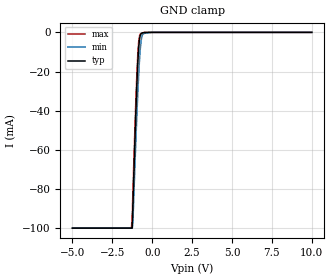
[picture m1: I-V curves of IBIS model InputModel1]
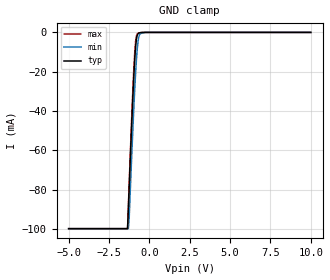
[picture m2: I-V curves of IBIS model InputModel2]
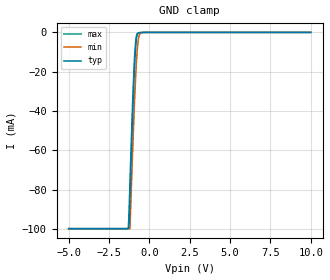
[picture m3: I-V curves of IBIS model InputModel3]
[IBIS Ver]   2.1
[File name]   ef008sa5.ibs   | e= TSOP f= Reverse Pinout,
|   | f0008sa= abbr chip name, 5= 5V Vcc
[File Rev]   2.00
[Date]   23-February-96
[Source]   File generated from lab measurements at Intel Corporation
[Notes]   Rev 2.00 All data was replaced by actual measurements
   performed in a lab.
[Disclaimer] INTEL DEVELOPER'S SOFTWARE LICENSE AGREEMENT
| BY USING THIS SOFTWARE, YOU ARE AGREEING TO BE BOUND
| BY THE TERMS OF THIS AGREEMENT.  DO NOT USE THE SOFTWARE
| UNTIL YOU HAVE CAREFULLY READ AND AGREED TO THE FOLLOWING
| TERMS AND CONDITIONS.  IF YOU DO NOT AGREE TO THE TERMS
| OF THIS AGREEMENT, PROMPTLY RETURN THE SOFTWARE PACKAGE
| AND ANY ACCOMPANYING ITEMS.
| IF YOU USE THIS SOFTWARE, YOU WILL BE BOUND BY THE TERMS
| OF THIS AGREEMENT
| LICENSE: Intel Corporation ("Intel") grants you the non-exclusive right
| to use the enclosed software program ("Software").  You will not use,
| copy, modify, rent, sell or transfer the Software or any portion
| thereof, except as provided in this Agreement.
| System OEM Developers may:
| 1.   Copy the Software for support, backup or archival purposes;
| 2.   Install, use, or distribute Intel owned Software in object code
|   only;
| 3.   Modify and/or use Software source code that Intel directly makes
|   available to you as an OEM Developer;
| 4.   Install, use, modify, distribute, and/or make or have made
|   derivatives ("Derivatives") of Intel owned Software under the
|   terms and conditions in this Agreement, ONLY if you are a System
|   OEM Developer and NOT an end-user.
| RESTRICTIONS:
| YOU WILL NOT:
| 1.   Copy the Software, in whole or in part, except as provided for
|   in this Agreement;
| 2.   Decompile or reverse engineer any Software provided in object
|   code format;
| 3.   Distribute any Software or Derivative code to any end-users,
|   unless approved by Intel in a prior writing.
| TRANSFER: You may transfer the Software to another OEM
| Developer if the receiving party agrees to the terms of this
| Agreement at the sole risk of any receiving party.
| OWNERSHIP AND COPYRIGHT OF SOFTWARE:
| Title to the Software and all copies thereof remain with Intel
| or its vendors.  The Software is copyrighted and is protected by
| United States and international copyright laws.  You will not
| remove the copyright notice from the Software.  You agree to
| prevent any unauthorized copying of the Software.
| DERIVATIVE WORK: OEM Developers that make or have made
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[Copyright]   Copyright 1996, Intel Corporation, All Rights Reserved
[Component]   F28F008SA   | 40-lead TSOP package, 28F008SA
[Manufacturer]  Intel   | Boot Block (tm)
|   | operating in 5V Vcc range
[Package]
|The following values apply for the leadframe.
|Variable   typ   min   max
R_pkg   135m   126m   144m
L_pkg   3.95nH   3.62nH   4.28nH
C_pkg   0.39pF   0.38pF   0.40pF
|*****************************Pin Definitions**********************************
[Pin]   signal_name   model_name   R_pin   L_pin   C_pin
  1   NC   InputModel5
  2   NC   InputModel5
  3   WE#   InputModel3
  4   OE#   InputModel3
  5   RYBY#   RYBYOutput
  6   DQ7   InputOutput
  7   DQ6   InputOutput
  8   DQ5   InputOutput
  9   DQ4   InputOutput
 10   VCC   POWER
 11   GND   GND
 12   GND   GND
 13   DQ3   InputOutput
 14   DQ2   InputOutput
 15   DQ1   InputOutput
 16   DQ0   InputOutput
 17   A00   InputModel1
 18   A01   InputModel1
 19   A02   InputModel1
 20   A03   InputModel1
 21   A04   InputModel2
 22   A05   InputModel2
 23   A06   InputModel2
 24   A07   InputModel2
 25   A08   InputModel2
 26   A09   InputModel2
 27   A10   InputModel2
 28   A11   InputModel2
 29   RP#   InputModel4
 30   VPP   POWER
 31   VCC   POWER
 32   CE#   InputModel3
 33   A12   InputModel2
 34   A13   InputModel2
 35   A14   InputModel2
 36   A15   InputModel2
 37   A16   InputModel2
 38   A17   InputModel2
 39   A18   InputModel2
 40   A19   InputModel2
|**********************Input Model 5***************************************
[Model]   InputModel5
Model_type   Input
|   For NC pins
Vinl = 0.8V
Vinh = 2.0V
| Variable   typ   min   max
C_comp   5.61p   NA   7.6p
[Voltage Range]   5.0V   4.5V   5.5V
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| Models and submodels in the file (7): InputModel1 (Input), InputModel2 (Input), InputModel3 (Input), InputModel4 (Input), InputModel5 (Input), InputOutput (I/O), RYBYOutput (Output)
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|**************************Input Model 1***************************************
[Model]   InputModel1
Model_type   Input
|   For A[3:0]
Vinl = 0.8V
Vinh = 2.0V
| Variable   typ   min   max
C_comp   5.61p   NA   7.6p
[Voltage Range]   5.0V   4.5V   5.5V
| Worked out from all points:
|   GND clamp passes 1 mA (typ) near -0.72 V on its own axis
[GND_clamp]
|Voltage I(typ)   I(min)   I(max)
-5V       -99.85mA   -99.84mA   -99.85mA
-1.3V     -99.85mA   -99.84mA   -99.85mA
-1.25V    -99.83mA   -99.84mA   -92.56mA
-1.2V     -85.91mA   -94.75mA   -78.96mA
-1.05V    -46.93mA   -60.78mA   -40.45mA
-950mV    -24.37mA   -39.94mA   -18.85mA
-850mV    -8.175mA   -22.06mA   -4.862mA
-800mV    -3.667mA   -14.55mA   -1.917mA
-700mV    -717.5uA   -4.645mA   -522.5uA
-600mV    -274uA     -1.047mA   -226.9uA
0V        0A         0A         0A
10V       0A         0A         0A
[POWER_clamp]
| Input buffer circuits of this product do not intrinsically
| require a [POWER_clamp] definition.  This zero current
| [POWER_clamp] is provided for compatibility with some ibis
| parsers.
|   Voltage  I(typ)   I(min)   I(max)
-5V       0A         0A         0A
-4.75V    0A         0A         0A
9.75V     0A         0A         0A
10V       0A         0A         0A
|**********************Input Model 2************************************
[Model]   InputModel2
Model_type   Input
|   For A[19:4]
Vinl = 0.8V
Vinh = 2.0V
| Variable   typ   min   max
C_comp   5.61p   NA   7.6p
[Voltage Range]   5.0V   4.5V   5.5V
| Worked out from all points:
|   GND clamp passes 1 mA (typ) near -0.73 V on its own axis
[GND_clamp]
|Voltage I(typ)   I(min)   I(max)
-5V       -99.84mA   -99.84mA   -99.84mA
-1.35V    -99.84mA   -99.84mA   -99.84mA
-1.3V     -90.06mA   -99.84mA   -88.39mA
-1.25V    -79.28mA   -94.68mA   -77.04mA
-1.1V     -48.07mA   -64.47mA   -44.59mA
-950mV    -20.49mA   -36.5mA    -16.5mA
-850mV    -7.244mA   -20.62mA   -4.445mA
-750mV    -1.356mA   -8.439mA   -748.5uA
-700mV    -613.5uA   -4.588mA   -433.7uA
-600mV    -217.8uA   -1.014mA   -177.9uA
-250mV    0A         0A         0A
10V       0A         0A         0A
[POWER_clamp]
| Input buffer circuits of this product do not intrinsically
| require a [POWER_clamp] definition.  This zero current
| [POWER_clamp] is provided for compatibility with some ibis
| parsers.
|   Voltage  I(typ)   I(min)   I(max)
-5V       0A         0A         0A
-4.75V    0A         0A         0A
9.75V     0A         0A         0A
10V       0A         0A         0A
|*********************Input Model 3**************************************
[Model]   InputModel3
Model_type   Input
|   For WE#, OE# & CE#
Vinl = 0.8V
Vinh = 2.0V
| Variable   typ   min   max
C_comp   5.61p   NA   7.6p
[Voltage Range]   5.0V   4.5V   5.5V
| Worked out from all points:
|   GND clamp passes 1 mA (typ) near -0.73 V on its own axis
[GND_clamp]
|Voltage I(typ)   I(min)   I(max)
-5V       -99.85mA   -99.84mA   -99.85mA
-1.3V     -99.85mA   -99.84mA   -99.85mA
-1.25V    -96.72mA   -99.84mA   -89.03mA
-1.2V     -83.27mA   -99.84mA   -75.92mA
-1.05V    -45.34mA   -63.96mA   -38.88mA
-950mV    -23.44mA   -41.82mA   -18.03mA
-900mV    -14.49mA   -31.8mA    -10.01mA
-850mV    -7.737mA   -22.92mA   -4.505mA
-750mV    -1.246mA   -8.932mA   -592.5uA
-650mV    -239.3uA   -2.195mA   -180.6uA
-500mV    -36.72uA   -152.6uA   -55.65uA
10V       0A         0A         0A
[POWER_clamp]
| Input buffer circuits of this product do not intrinsically
| require a [POWER_clamp] definition.  This zero current
| [POWER_clamp] is provided for compatibility with some ibis
| parsers.
|   Voltage  I(typ)   I(min)   I(max)
-5V       0A         0A         0A
-4.75V    0A         0A         0A
9.75V     0A         0A         0A
10V       0A         0A         0A
